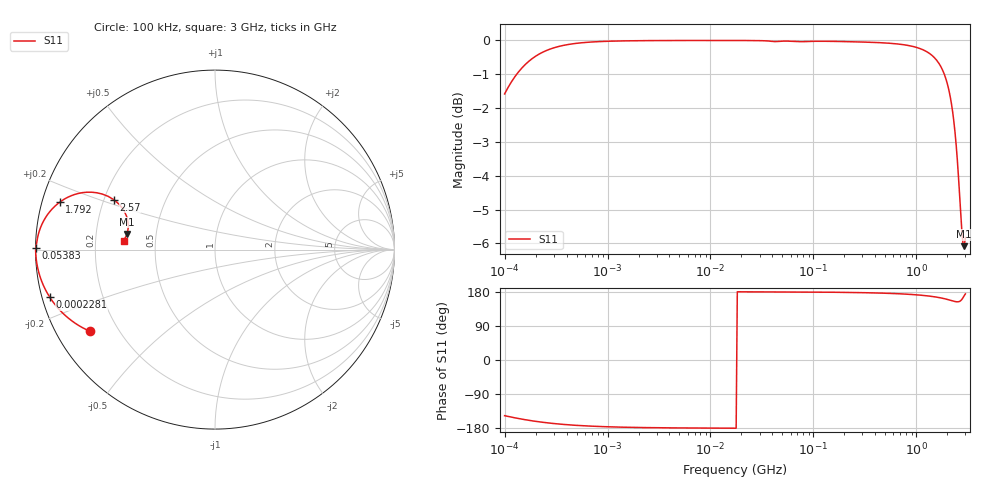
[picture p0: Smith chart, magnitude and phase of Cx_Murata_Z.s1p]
!Murata Part Number: GA255DR7E2104MW01
!X7R ceramic capacitor, package code size 2220, 250 Vac, 100 nF +/-20%, -55°c to 125°c
!Impedance provided by the manufacturer
# Hz S RI R 50
!Freq.(Hz) S11(Real) S11(Imag)
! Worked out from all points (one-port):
!   401 points, 100 kHz to 3 GHz, reference 50 ohm
!   lowest |S11| = -6.1 dB at 2.924 GHz (marker M1), VSWR 2.97, Z = 16.9 + j3.94 ohm
!   |S11| at or under -10 dB: nowhere
!   S11 on the Smith chart (normalised r, x): 100 kHz: 0.10, -0.29; 228.1 kHz: 0.02, -0.14; 53.83 MHz: 0.00, +0.00; 1.792 GHz: 0.05, +0.15; 2.57 GHz: 0.24, +0.22; 3 GHz: 0.32, +0.04
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100000  -0.6984 -0.4544
116723.1  -0.7583 -0.4234
151037.5  -0.8387 -0.3629
185621.1  -0.8862 -0.3126
228123.3  -0.9209 -0.2648
362777.3  -0.9661 -0.1752
656258  -0.9885 -0.0994
1316074  -0.9964 -0.05
2320182  -0.9984 -0.0282
4774418  -0.9992 -0.0131
1.732051e7  -0.9993 -0.00037
5.383243e7  -0.9972 0.00735
6.283488e7  -0.9964 0.00929
2.279507e8  -0.9946 0.0306
4.690719e8  -0.9895 0.0617
8.269535e8  -0.9765 0.1104
1.070062e9  -0.962 0.1459
1.315078e9  -0.9404 0.1842
1.575075e9  -0.9065 0.2273
1.7917e9  -0.8656 0.2639
2.038117e9  -0.7987 0.3011
2.259438e9  -0.7142 0.3197
2.441062e9  -0.6278 0.3094
2.570185e9  -0.5636 0.278
2.706139e9  -0.5072 0.218
2.776789e9  -0.4891 0.1772
2.923671e9  -0.4886 0.0876
3e9  -0.5089 0.0496
